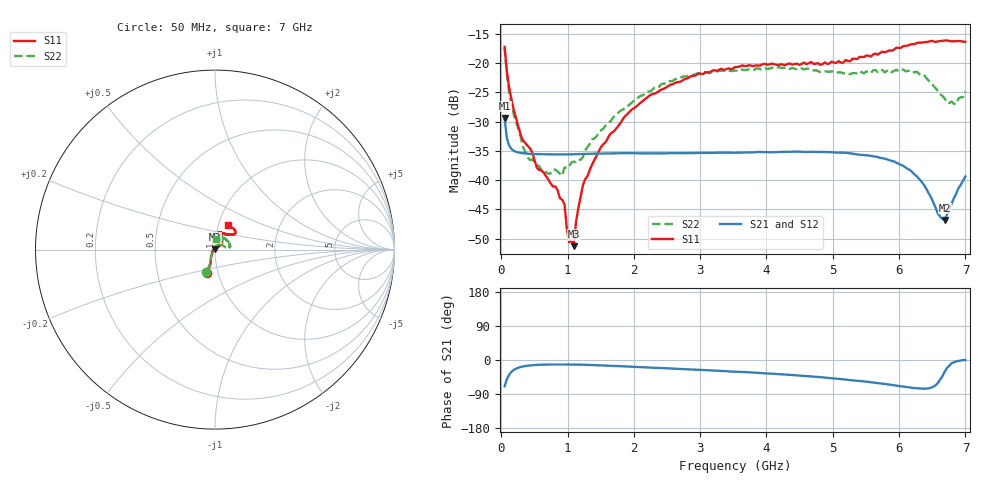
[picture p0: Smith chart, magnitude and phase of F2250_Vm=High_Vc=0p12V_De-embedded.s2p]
! Integrated Device Technology
! Corporate Headquarters
! 6024 Silver Creek Valley Road
! San Jose, CA 95138  USA
! Phone:  1-408-284-8200
! Toll Free:  1-800-223-1366
! Webpage:  http://www.idt.com/
! Timing and RF Division
! 515 Groton Road, Suite 102
! Westford, MA 01886-6024
! Device:  F2250
! Description: Voltage Variable RF Attenuator
! Frequency:  50.0 -  6000.00 MHz
! Package:  3x3 mm Thin QFN Plastic Package: 16 pin
! Ports:  2 RF, 3 DC
!  Pin  1  = GND
!  Pin  2  = NC
!  Pin  3  = RF1  = Port 1
!  Pin  4  = NC
!  Pin  5  = GND
!  Pin  6  = GND
!  Pin  7  = GND
!  Pin  8  = GND
!  Pin  9  = NC
!  Pin 10  = RF2  = Port 2
!  Pin 11  = NC
!  Pin 12  = GND
!  Pin 13  = GND
!  Pin 14  = VCNTRL
!  Pin 15  = VDD
!  Pin 16  = VMODE
! Vcntrl:  0.120 Volts
! Vmode:  +3.300 Volts
! Vdd:  +3.30  Volts
! Current:  1.240 mA
! Data:  The device was measured on a the F2250 evaluation board which has
!  individual transmission lines to the RF pins.  Data was collected
!  using a calibrated network analyzer.  The evaluation board was
!  de-embedded using a TRL calibration technique.
!  The reference plane is the edge of the package pin.
! Misc:  SN 10
!  Action Tracker AT0258
! Date Measured:  2014-11-26
! Date:  2015-10-15  MJV
! Note:
!  Integrated Device Technology supplies this data as a sample of measured
!  data at the package pin for this product.  Your particular data for this
!  product may vary.
!  Data was taken at 25 degrees C.
!  Integrated Device Technology reserves the right to change this data at anytime.
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# GHz S dB R 50
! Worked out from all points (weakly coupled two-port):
!   201 points, 50 MHz to 7 GHz, reference 50 ohm
!   highest |S21| = -29.38 dB at 50 MHz (marker M1); lowest = -46.8 dB at 6.687 GHz (marker M2)
!   lowest |S11| = -51.3 dB at 1.093 GHz (marker M3), VSWR 1.01, Z = 50 + j0.272 ohm
!   |S11| at or under -10 dB: start of sweep to end of sweep
!   |S22| runs from -39.2 to -17.4 dB; largest |S21 - S12| = 6.4e-05
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0.05  -17.18 -108.5  -29.38 -69.5  -29.38 -69.5  -17.37 -110.6
0.08475  -21.47 -107.4  -32.86 -50.1  -32.86 -50.0  -21.87 -109.0
0.15425  -26.23 -116.6  -34.68 -31.0  -34.68 -31.0  -27.10 -120.7
0.29325  -32.28 -127.5  -35.35 -18.5  -35.35 -18.5  -32.65 -133.5
0.3975  -34.12 -142.3  -35.48 -15.1  -35.48 -15.1  -36.08 -158.5
0.5365  -37.87 -154.5  -35.55 -12.9  -35.55 -12.9  -37.49 -179.9
0.64075  -38.75 -162.5  -35.58 -12.2  -35.58 -12.2  -38.90 160.6
0.91875  -43.36 155.8  -35.60 -11.8  -35.60 -11.8  -39.21 127.8
0.9535  -44.16 171.0  -35.60 -11.8  -35.60 -11.8  -37.82 124.3
1.023  -50.64 140.6  -35.59 -11.9  -35.59 -11.9  -37.70 108.0
1.0925  -51.30 89.0  -35.58 -12.0  -35.58 -12.0  -36.84 98.6
1.12725  -47.13 61.8  -35.56 -12.1  -35.56 -12.1  -36.91 91.8
1.2315  -40.85 41.1  -35.52 -12.4  -35.52 -12.5  -36.06 77.3
1.6485  -32.02 41.3  -35.43 -15.2  -35.44 -15.2  -29.91 60.0
2.37825  -24.76 46.7  -35.40 -21.0  -35.40 -21.1  -24.03 53.9
3.525  -20.65 71.8  -35.31 -30.6  -35.32 -30.7  -21.26 72.9
4.7065  -20.07 72.0  -35.15 -43.9  -35.15 -43.9  -21.21 70.3
5.85325  -17.79 40.5  -36.58 -64.8  -36.58 -64.9  -21.13 23.3
6.27025  -16.53 39.4  -39.38 -74.4  -39.40 -74.5  -21.46 8.6
6.68725  -16.11 47.9  -46.80 -31.0  -46.77 -30.7  -26.03 28.5
6.861  -16.21 54.5  -42.31 -3.7  -42.27 -3.7  -26.96 57.4
7  -16.32 62.4  -39.36 -0.1  -39.32 -0.3  -24.82 83.6
